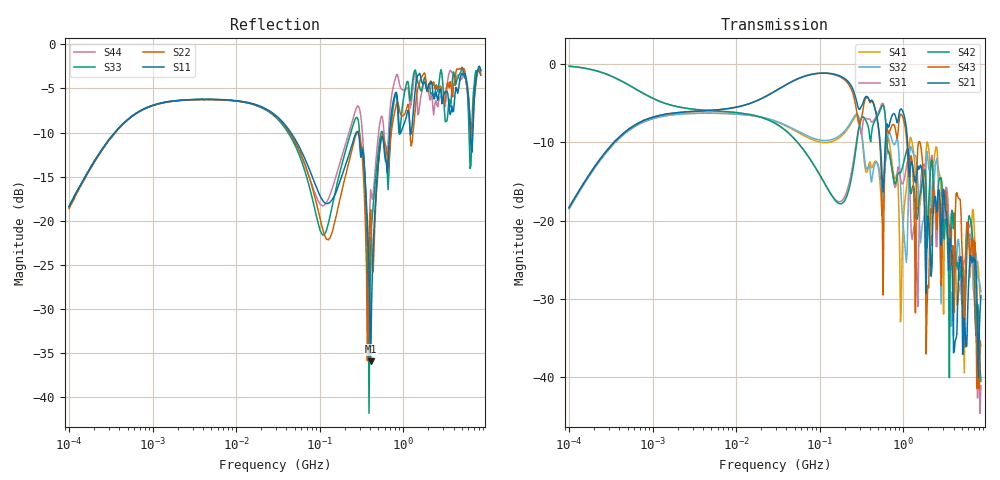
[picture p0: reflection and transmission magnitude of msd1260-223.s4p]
# MHz S MA R 50
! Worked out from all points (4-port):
!   498 points, 100 kHz to 8.5 GHz, reference 50 ohm
!   strongest paths, dB at 100 kHz, 1.698 MHz, 29.49 MHz, 500.7 MHz, 8.5 GHz:
!     S21: -18.3, -6.3, -3.4, -7.7, -29.6
!     S43: -18.3, -6.3, -3.4, -7.9, -35.9
!     S42: -0.3, -5.3, -7.6, -6.5, -40.5
!     S31: -0.3, -5.3, -7.6, -6.2, -41.1
!     S32: -18.5, -6.5, -7.3, -12.8, -29.1
!     S41: -18.5, -6.5, -7.3, -13.1, -29.8
!   lowest |S11| = -36.0 dB at 407.6 MHz (marker M1), VSWR 1.03, Z = 49.2 + j1.36 ohm
!   |S11| at or under -10 dB: 45.21 MHz to 274.3 MHz (229.1 MHz wide, 143 % of centre); 286.8 MHz to 686.7 MHz (399.9 MHz wide, 82.2 % of centre); 6.366 GHz to 6.82 GHz (454 MHz wide, 6.89 % of centre)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
0.1  0.1207 74.1  0.1217 74.3  0.9683 -7.0  0.1195 -105.8
     0.1217 74.3  0.117 74.9  0.1194 -105.9  0.97 -6.9
     0.9683 -7.0  0.1194 -105.9  0.1193 74.4  0.1217 74.2
     0.1195 -105.8  0.97 -6.9  0.1217 74.2  0.1201 74.7
276.4819  0.3182 -36.6  0.5781 -66.6  0.3267 103.6  0.4666 -9.8
          0.5781 -66.6  0.3143 -24.5  0.4812 -14.7  0.3103 113.4
          0.3267 103.6  0.4812 -14.7  0.3857 -33.6  0.501 -75.6
          0.4666 -9.8  0.3103 113.4  0.501 -75.6  0.4383 -28.5
407.6417  0.0159 119.8  0.5809 -78.6  0.4352 -0.5  0.2286 -41.4
          0.5809 -78.6  0.1154 -17.2  0.1888 -49.4  0.3196 3.9
          0.4352 -0.5  0.1888 -49.4  0.07066 47.8  0.5691 -82.1
          0.2286 -41.4  0.3196 3.9  0.5691 -82.1  0.1502 23.1
1336.696  0.4492 -104.7  0.1995 172.9  0.09007 -149.0  0.2694 -147.8
          0.1995 172.9  0.3482 -107.0  0.2645 -144.3  0.1652 -136.5
          0.09007 -149.0  0.2645 -144.3  0.6844 -120.7  0.1502 130.5
          0.2694 -147.8  0.1652 -136.5  0.1502 130.5  0.6304 -126.8
2840.13  0.5288 100.8  0.06968 20.1  0.07512 42.1  0.1551 4.6
         0.06968 20.1  0.5733 105.7  0.02939 89.9  0.188 19.9
         0.07512 42.1  0.02939 89.9  0.7184 97.0  0.03875 55.1
         0.1551 4.6  0.188 19.9  0.03875 55.1  0.5048 115.9
4802.421  0.6451 -85.9  0.05873 132.3  0.05245 -124.1  0.03988 -94.4
          0.05873 132.3  0.7308 -88.5  0.05593 -117.0  0.04474 -104.9
          0.05245 -124.1  0.05593 -117.0  0.6867 -84.6  0.1368 103.9
          0.03988 -94.4  0.04474 -104.9  0.1368 103.9  0.6236 -90.9
8500  0.7144 -57.2  0.03321 -37.7  0.008828 -3.8  0.03232 -141.0
      0.03321 -37.7  0.6813 -57.3  0.03521 -140.6  0.009433 -75.8
      0.008828 -3.8  0.03521 -140.6  0.6679 -48.4  0.01596 -52.4
      0.03232 -141.0  0.009433 -75.8  0.01596 -52.4  0.7034 -56.3
